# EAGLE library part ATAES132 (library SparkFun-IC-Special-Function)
Crypto 32Kb Serial EEPROM AES-128-CCM MAC Secure Storage for 128-bit keys Encrypted User Memory Readn and Write HWRNG 2.5V to 5.5V Datasheet SparkFun Products CryptoCape (DEV-12773) SparkFun CryptoShield (DEV-13183)
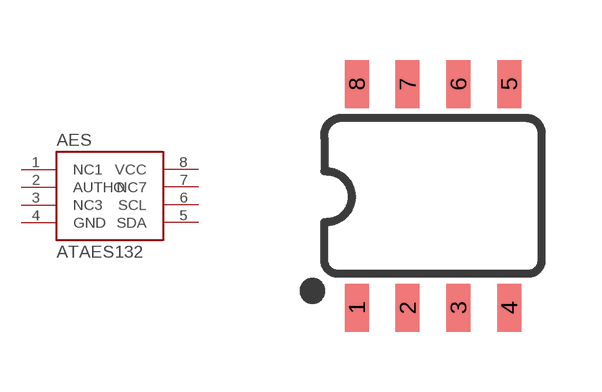
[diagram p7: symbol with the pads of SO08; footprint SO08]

Designator prefix AES

## ATAES132 (PROD_ID: IC-11983; VALUE: ATAES132)  [SO08]
1  NC1  nc
2  AUTHO
3  NC3  nc
4  GND  pwr
5  SDA
6  SCL
7  NC7  nc
8  VCC  pwr

## Footprint SO08 (pad centres in mm)
SOIC, 0.15 inch width
smd 0.6 x 1.2: 1 -1.905,-2.8; 2 -0.635,-2.8; 3 0.635,-2.8; 4 1.905,-2.8; 5 1.905,2.8; 6 0.635,2.8; 7 -0.635,2.8; 8 -1.905,2.8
